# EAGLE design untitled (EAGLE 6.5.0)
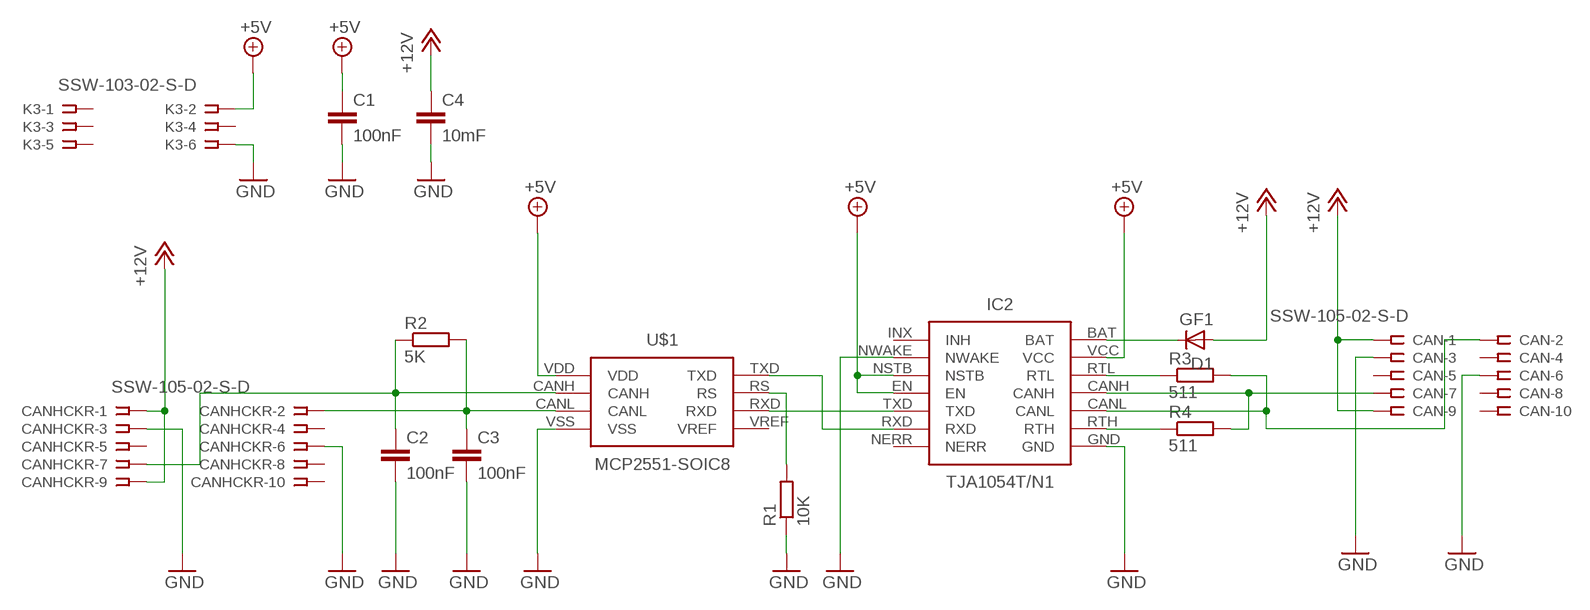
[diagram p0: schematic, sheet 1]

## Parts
C1  100nF  C-EUC0805  [C0805]
C2  100nF  C-EUC0805  [C0805]
C3  100nF  C-EUC0805  [C0805]
C4  10mF  C-EUC0805  [C0805]
CAN  SSW-105-02-S-D  [SSW-105-02-S-D]
CANHCKR  SSW-105-02-S-D  [SSW-105-02-S-D]
D1  GF1  [SMA-DO214AC]
IC2  TJA1054T/N1  [TJA1054T/N1]
K3  SSW-103-02-S-D  [SSW-103-02-S-D]
R1  10K  R-EU_M0805  [M0805]
R2  5K  R-EU_M0805  [M0805]
R3  511  R-EU_M0805  [M0805]
R4  511  R-EU_M0805  [M0805]
U$1  MCP2551-SOIC8  [MCP2551-SOIC8]

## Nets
+5V: C1.1 IC2.EN IC2.NSTB IC2.VCC K3.2 U$1.VDD
+12V: C4.1 CAN.1 CAN.9 CANHCKR.1 CANHCKR.9 D1.A
GND: C1.2 C2.2 C3.2 C4.2 CAN.3 CAN.6 CANHCKR.3 CANHCKR.6 IC2.GND IC2.NWAKE K3.6 R1.1 U$1.VSS
N$1: IC2.TXD U$1.RXD
N$2: IC2.RXD U$1.TXD
N$3: R1.2 U$1.RS
N$4: C2.1 CANHCKR.7 R2.1 U$1.CANH
N$5: C3.1 CANHCKR.2 R2.2 U$1.CANL
N$6: IC2.RTL R3.1
N$7: CAN.7 IC2.CANH R4.2
N$8: CAN.2 IC2.CANL R3.2
N$9: IC2.RTH R4.1
N$10: D1.K(C) IC2.BAT
Unconnected: CAN.4 CAN.5 CAN.8 CAN.10 CANHCKR.4 CANHCKR.5 CANHCKR.8 CANHCKR.10 IC2.INX(INH) IC2.NERR K3.1 K3.3 K3.4 K3.5 U$1.VREF

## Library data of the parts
C1-C4 = resistor:C-EU: CAPACITOR, European symbol
CAN CANHCKR = con-samtec:SSW-105-02-S-D: THROUGH-HOLE .025" SQ POST SOCKET Source: Samtec SSW.pdf; MPN: SSW-105-02-S-D; OC_FARNELL: unknown; OC_NEWARK: 11P9398
D1 = diode:GF1: DIODE
IC2 = can-adapter:TJA1054T/N1
K3 = con-samtec:SSW-103-02-S-D: THROUGH-HOLE .025" SQ POST SOCKET Source: Samtec SSW.pdf; MPN: SSW-103-02-S-D; OC_FARNELL: unknown; OC_NEWARK: 11P9365
R1-R4 = resistor:R-EU_: RESISTOR, European symbol
U$1 = can-adapter:MCP2551-SOIC8

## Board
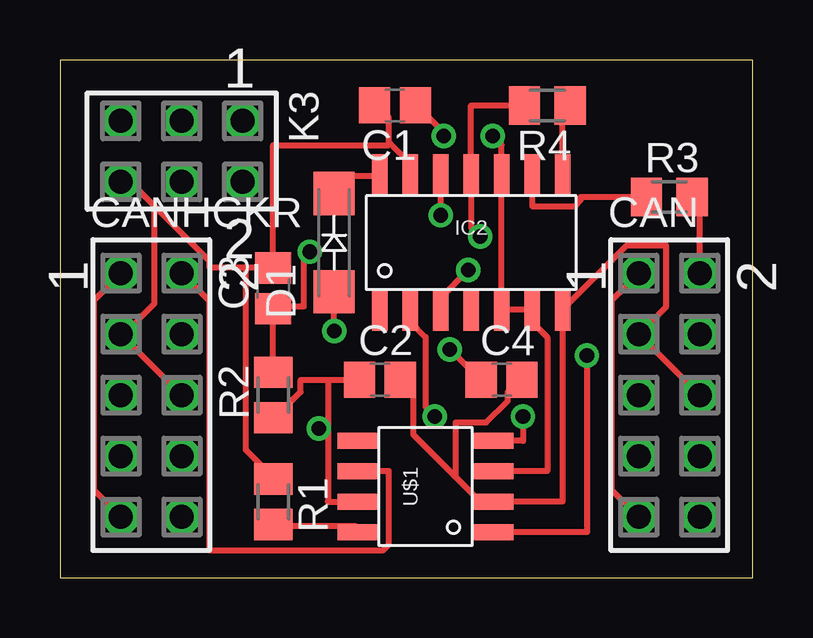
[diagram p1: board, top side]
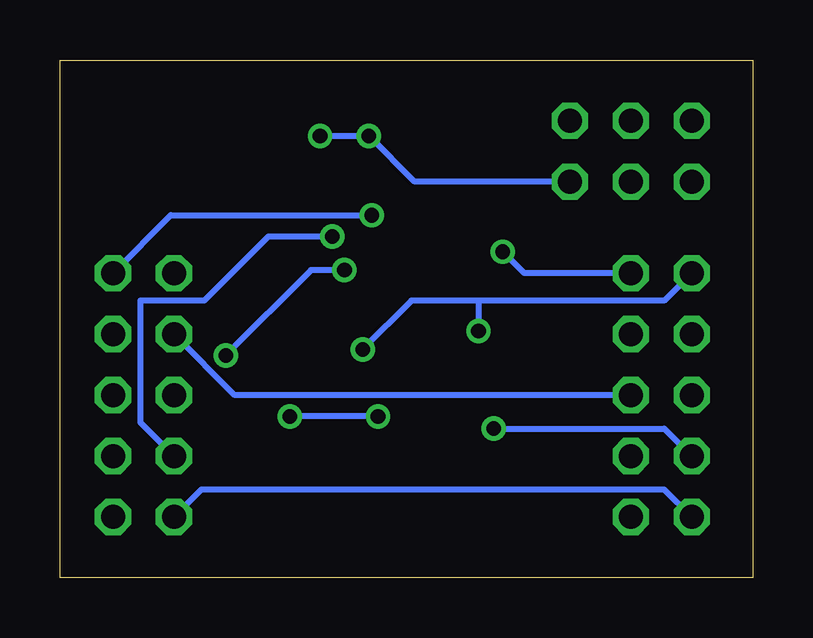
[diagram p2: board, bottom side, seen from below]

Size 28.88 x 21.58 mm. Coordinates in mm from the lower left corner, seen from the top.
Outline: 0,0 28.88,0 28.88,21.58 0,21.58 0,0
Copper layers (1*16): Top 0.035mm / dielectric 1.5mm / Bottom 0.035mm
Design rules "default": minimum track width 10mil, minimum drill 24mil, track to track 8mil, track to pad 8mil, pad to pad 8mil, via to via 8mil, smd to smd 8mil, copper to edge 40mil, drill to drill 8mil, minimum pad ring 10mil, minimum via ring 8mil, stop-mask expansion 4mil, vias tented up to drill 0mil, thermal gap 10mil

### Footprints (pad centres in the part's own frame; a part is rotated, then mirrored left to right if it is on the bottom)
C0805 = smd 1.3 x 1.5: 1 -0.85,0; 2 0.85,0
SSW-105-02-S-D = drill 1 pad 1.5 octagon: 1 -5.08,-1.27; 2 -5.08,1.27; 3 -2.54,-1.27; 4 -2.54,1.27; 5 0,-1.27; 6 0,1.27; 7 2.54,-1.27; 8 2.54,1.27; 9 5.08,-1.27; 10 5.08,1.27
SMA-DO214AC = smd 1.8 x 1.7: A -2.05,0; K 2.05,0
TJA1054T/N1 = smd 0.65 x 1.75: BAT -3.81,2.8; CANH 0,2.8; CANL -1.27,2.8; EN 2.54,-2.8; GND -2.54,2.8; INX -3.81,-2.8; NERR 0,-2.8; NSTB 1.27,-2.8; NWAKE 3.81,-2.8; RTH 3.81,2.8; RTL 2.54,2.8; RXD -1.27,-2.8; TXD -2.54,-2.8; VCC 1.27,2.8
SSW-103-02-S-D = drill 1 pad 1.5 octagon: 1 -2.54,-1.27; 2 -2.54,1.27; 3 0,-1.27; 4 0,1.27; 5 2.54,-1.27; 6 2.54,1.27
M0805 = smd 1.3 x 1.6: 1 -0.95,0; 2 0.95,0
MCP2551-SOIC8 = smd 0.65 x 1.75: CANH -0.635,2.8; CANL 0.635,2.8; RS -1.905,2.8; RXD 1.905,-2.8; TXD -1.905,-2.8; VDD 0.635,-2.8; VREF 1.905,2.8; VSS -0.635,-2.8

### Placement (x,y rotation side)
C1  13.97,19.68 180 top
C2  13.34,8.26 0 top
C3  8.89,12.06 90 top
C4  18.41,8.26 0 top
CAN  25.4,7.62 270 top
CANHCKR  3.81,7.62 270 top
D1  11.43,13.97 90 top
IC2  17.14,13.97 0 top
K3  5.08,17.78 180 top
R1  8.89,3.17 270 top
R2  8.89,7.62 90 top
R3  25.4,15.88 0 top
R4  20.32,19.68 180 top
U$1  15.24,3.81 90 top

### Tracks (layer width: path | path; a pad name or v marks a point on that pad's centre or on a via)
+5V  (via drill 0.61)
  Top 0.254: v16,18.41 16,18.54 14.86,19.68 C1.1 | U$1.VDD 20.32,4.45 20.32,10.03 19.68,10.67 IC2.EN IC2.NSTB | IC2.NSTB IC2.VCC 18.41,18.03 v18.03,18.41 | IC2.NSTB
  Bottom 0.254: K3.2 14.1,16.51 v16,18.41 v18.03,18.41
+12V  (via drill 0.61)
  Top 0.254: CAN.9 22.99,3.68 22.99,11.56 CAN.1 | v16.26,9.53 17.53,8.26 C4.1 | v11.43,10.29 D1.A | CANHCKR.9 1.4,3.68 1.4,11.56 CANHCKR.1
  Bottom 0.254: v16.26,9.53 14.22,11.56 11.43,11.56 | 11.43,11.56 3.68,11.56 CANHCKR.1 | 11.43,11.56 v11.43,10.29 | CAN.9 22.99,3.68 3.68,3.68 CANHCKR.9
GND
  Top 0.254: 16.45,4.25 17.53,3.17 U$1.VSS 20.95,3.17 IC2.NWAKE 23.62,13.84 25.27,13.84 25.27,11.3 CAN.3 24.26,10.16 24.26,10.03 CAN.6 | 16.45,4.25 14.73,5.97 14.73,7.75 14.22,8.26 C2.2 | C4.2 19.18,8.26 18.67,7.75 18.67,7.37 17.78,6.48 16.51,6.48 16.51,4.32 16.45,4.25 | CANHCKR.6 CANHCKR.3 2.67,10.16 3.94,11.43 3.94,15.37 4,15.43 | 13.78,18.1 14.61,17.27 IC2.GND | 13.78,18.1 13.72,18.16 13.72,19.18 13.21,19.68 C1.2 | 7.75,12.95 6.22,12.95 6.22,13.21 4,15.43 | 7.75,12.95 8.89,12.95 | 4,15.43 2.92,16.51 K3.6 | 7.75,12.95 7.75,5.33 8.89,4.19 R1.1 | 8.89,12.95 8.89,18.03 13.72,18.03 13.78,18.1 | 8.89,12.95 C3.2
  Bottom 0.254: CAN.3 21.59,7.62 CANHCKR.6
N$1  (via drill 0.61)
  Top 0.254: U$1.RXD 19.3,5.71 v19.3,6.73 | v15.62,6.73 15.24,7.11 15.24,10.03 14.61,10.67 IC2.TXD
  Bottom 0.254: v15.62,6.73 v19.3,6.73
N$2  (via drill 0.61)
  Top 0.254: U$1.TXD 21.97,1.91 v21.97,9.27 | v17.02,12.83 15.88,11.68 IC2.RXD
  Bottom 0.254: v21.97,9.27 18.41,12.83 v17.02,12.83
N$3
  Top 0.254: R1.2 8.89,2.16 12.32,2.16 12.32,1.91 U$1.RS
N$4  (via drill 0.61)
  Top 0.254: 11.18,8.26 10.03,8.26 10.03,7.75 8.89,6.6 R2.1 | 11.18,8.26 C2.1 | U$1.CANH 11.18,3.17 11.18,6.22 | 11.18,8.26 11.18,6.22 | 11.18,6.22 v10.79,6.22
  Bottom 0.254: CANHCKR.7 3.68,6.22 v10.79,6.22
N$5  (via drill 0.61)
  Top 0.254: R2.2 C3.1 8.89,11.3 10.16,11.3 10.16,13.34 v10.41,13.59 | U$1.CANL 13.72,4.45 13.72,1.4 13.46,1.14 6.22,1.14 6.22,11.56 CANHCKR.2
  Bottom 0.254: v10.41,13.59 9.53,12.7 CANHCKR.2
N$6
  Top 0.254: R3.1 21.72,15.88 21.72,15.75 21.46,15.49 19.68,15.49 IC2.RTL
N$7  (via drill 0.61)
  Top 0.254: R4.2 17.14,19.68 IC2.CANH 17.14,14.61 v17.53,14.22
  Bottom 0.254: CAN.7 25.53,6.48 25.53,11.56 22.86,11.56 20.19,14.22 v17.53,14.22
N$8  (via drill 0.61)
  Top 0.254: CAN.2 26.67,15.62 26.42,15.88 R3.2 | v15.88,15.11 IC2.CANL
  Bottom 0.254: v15.88,15.11 24.26,15.11 CAN.2
N$9
  Top 0.254: IC2.RTH 20.95,19.43 21.21,19.68 R4.1
N$10
  Top 0.254: D1.K 11.43,16.76 IC2.BAT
